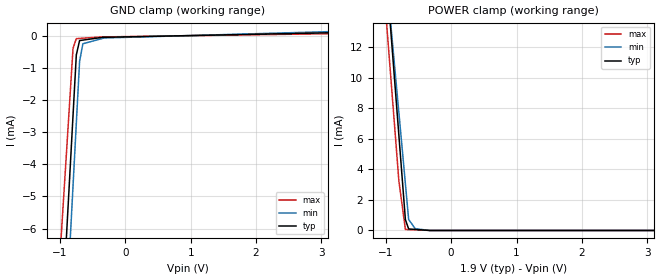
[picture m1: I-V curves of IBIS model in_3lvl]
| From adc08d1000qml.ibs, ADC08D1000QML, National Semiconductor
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[Model] in_3lvl
Model_type Input
Vinl = 290.000mV
Vinh = 1.62000V
C_comp 630.000fF 630.000fF 630.000fF
| variable typ   min   max
[Voltage Range] 1.90000V 1.80000V 2.00000V
[POWER Clamp Reference] 1.90000V 1.80000V 2.00000V
[GND Clamp Reference] 0.00000V 0.00000V 0.00000V
[Temperature Range]   25   125   -55
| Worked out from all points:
|   GND clamp passes 1 mA (typ) near -0.76 V on its own axis
|   POWER clamp passes 1 mA (typ) near -0.71 V on its own axis
[GND Clamp]
-1.9V     -43.64mA   -47.14mA   -35.9mA
-800mV    -2.472mA   -4.664mA   -392.4uA
-750mV    -600.6uA   -2.734mA   -93.98uA
-700mV    -153.6uA   -802.9uA   -86.99uA
-650mV    -139.3uA   -254uA     -79.99uA
-375mV    -60.99uA   -100.7uA   -41.51uA
-350mV    -53.87uA   -86.78uA   -40.79uA
-325mV    -52.84uA   -72.84uA   -40.07uA
3.8V      116.3uA    162.8uA    78.79uA
[POWER Clamp]
-1.9V     67.26mA    59.22mA    63.78mA
-850mV    9.027mA    10.08mA    6.011mA
-800mV    6.254mA    7.74mA     3.26mA
-700mV    708.6uA    3.06mA     64.65uA
-650mV    100.4uA    720.5uA    56.57uA
-550mV    69.51uA    120uA      40.41uA
-500mV    54.06uA    90uA       32.32uA
-400mV    23.17uA    38.57uA    16.16uA
-325mV    0A         0A         4.041uA
-250mV    0A         0A         0A
3.8V      0A         0A         0A
